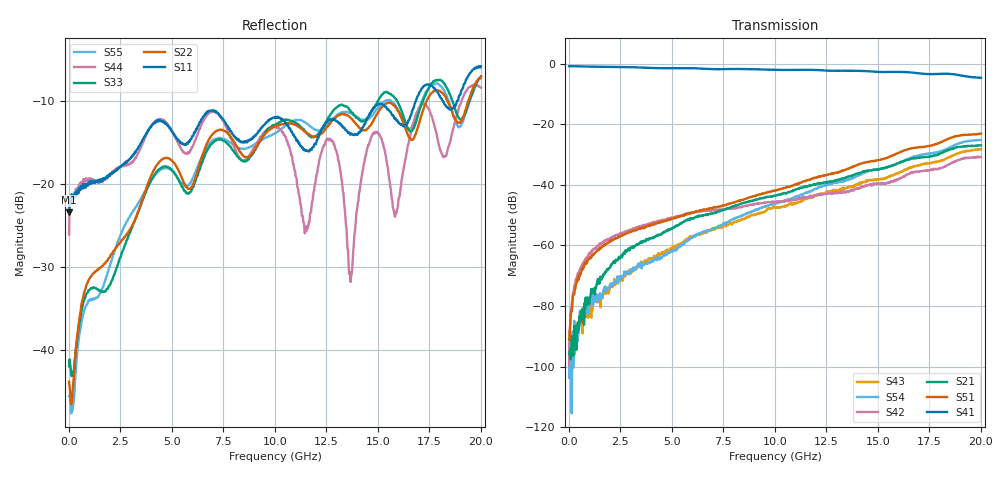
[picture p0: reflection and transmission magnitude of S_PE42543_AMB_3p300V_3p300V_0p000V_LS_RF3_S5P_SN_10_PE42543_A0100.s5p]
!Agilent Technologies,N5230C,MY49001593,A.09.33.09
!Agilent N5230C: A.09.33.09
!Date: Friday, March 21, 2014 07:23:38
!Correction: S11(Full 5 Port(1,2,3,5,6))
!S12(Full 5 Port(1,2,3,5,6))
!S13(Full 5 Port(1,2,3,5,6))
!S15(Full 5 Port(1,2,3,5,6))
!S16(Full 5 Port(1,2,3,5,6))
!S21(Full 5 Port(1,2,3,5,6))
!S22(Full 5 Port(1,2,3,5,6))
!S23(Full 5 Port(1,2,3,5,6))
!S25(Full 5 Port(1,2,3,5,6))
!S26(Full 5 Port(1,2,3,5,6))
!S31(Full 5 Port(1,2,3,5,6))
!S32(Full 5 Port(1,2,3,5,6))
!S33(Full 5 Port(1,2,3,5,6))
!S35(Full 5 Port(1,2,3,5,6))
!S36(Full 5 Port(1,2,3,5,6))
!S51(Full 5 Port(1,2,3,5,6))
!S52(Full 5 Port(1,2,3,5,6))
!S53(Full 5 Port(1,2,3,5,6))
!S55(Full 5 Port(1,2,3,5,6))
!S56(Full 5 Port(1,2,3,5,6))
!S61(Full 5 Port(1,2,3,5,6))
!S62(Full 5 Port(1,2,3,5,6))
!S63(Full 5 Port(1,2,3,5,6))
!S65(Full 5 Port(1,2,3,5,6))
!S66(Full 5 Port(1,2,3,5,6))
!S5P File: Measurements: <S11,S12,S13,S15,S16>,
!<S21,S22,S23,S25,S26>,
!<S31,S32,S33,S35,S36>,
!<S51,S52,S53,S55,S56>,
!<S61,S62,S63,S65,S66>:
# Hz S  dB  R 50
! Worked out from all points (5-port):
!   801 points, 10 MHz to 20 GHz, reference 50 ohm
!   strongest paths, dB at 10 MHz, 5.008 GHz, 10.01 GHz, 15 GHz, 20 GHz:
!     S41: -0.8, -1.4, -2.0, -2.7, -4.6
!     S51: -91.1, -51.3, -41.9, -31.8, -23.1
!     S21: -95.8, -54.5, -43.6, -35.0, -26.9
!     S42: -99.4, -51.0, -45.7, -39.4, -30.8
!     S54: -103.7, -61.9, -46.1, -34.8, -25.2
!     S43: -88.3, -60.7, -47.2, -38.2, -28.2
!   lowest |S11| = -23.4 dB at 10 MHz (marker M1), VSWR 1.14, Z = 56.8 - j2.28 ohm
!   |S11| at or under -10 dB: start of sweep to 16.85 GHz; 18.14 GHz to 18.88 GHz (741.8 MHz wide, 4.01 % of centre)
